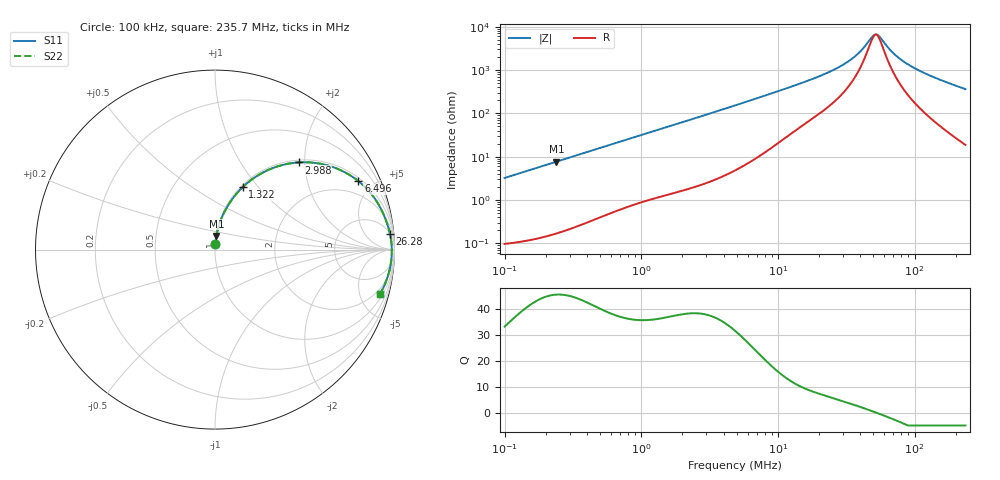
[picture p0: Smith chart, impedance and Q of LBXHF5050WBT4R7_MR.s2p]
! LBXHF5050WBT4R7_MR  S-PARAMETER MODEL  ( General Type )
! Model Generated by TAIYO YUDEN Corporation (http://www.ty-top.com)
! Version 1.0
! TAIYO YUDEN Control No. 210719NI43SB-FBB
! Copyright(c) 2021 TAIYO YUDEN CO.,LTD. All Rights Reserved.
! Product Description (link to TY-COMPAS)
! https://ds.yuden.co.jp/TYCOMPAS/or/detail?pn=LBXHF5050WBT4R7MMR&u=M
! Products Name : Inductors
! Characteristics :
!  Inductance : 4.7 uH , SRF(min) : 35 MHz , DC Resistance(max) : 0.0696 Ohm
!  Rated Current : Saturation :2100 mA , Temp Rise : 1500 mA
!  Case Size : 5.0 x 5.0 / 0.197 x 0.197 [mm/inch] , Thickness : 2.2 / 0.087 [mm/inch]
!  (Conditions: Temperature = 25 degC , DC Bias Current/Voltage = 0A / 0V)
! External Node Assignments :
!  1  o---GGG---o  2
! GND o---------o GND
! Frequency Range : 0.1MHz  -  235.669543MHz  [ 402 STEP ]
# MHz S RI R 50
! Freq[MHz].  S11 Real  S11 Imag  S21 Real  S21 Imag  S12 Real  S12 Imag  S22 Real  S22 Imag
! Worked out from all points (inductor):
!   401 points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, 100 kHz to 235.7 MHz, reference 50 ohm
!   read as one part in series: L = 5.14 uH near 104 kHz
!   highest Q = 45.6 at 239.5 kHz (marker M1), where L = 5.13 uH
!   self-resonance near 51.84 MHz
!   S11 on the Smith chart (normalised r, x): 100 kHz: 1.00, +0.06; 1.322 MHz: 1.02, +0.83; 2.988 MHz: 1.05, +1.87; 6.496 MHz: 1.16, +4.11; 26.28 MHz: 5, +21; 235.7 MHz: 1.38, -7.25
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0.1  0.00201 0.0322  0.998 -0.0322  0.998 -0.0322  0.00201 0.0322
0.239543  0.00758 0.0765  0.9924 -0.0765  0.9924 -0.0765  0.00758 0.0765
0.367165  0.0163 0.1157  0.9837 -0.1157  0.9837 -0.1157  0.0163 0.1157
0.767767  0.0617 0.2272  0.9383 -0.2272  0.9383 -0.2272  0.0617 0.2272
1.322181  0.154 0.3474  0.846 -0.3474  0.846 -0.3474  0.154 0.3474
1.348099  0.1588 0.352  0.8412 -0.352  0.8412 -0.352  0.1588 0.352
1.949423  0.2761 0.4341  0.7239 -0.4341  0.7239 -0.4341  0.2761 0.4341
2.988015  0.4662 0.4858  0.5338 -0.4858  0.5338 -0.4858  0.4662 0.4858
4.854581  0.6933 0.4456  0.3067 -0.4456  0.3067 -0.4456  0.6933 0.4456
6.495508  0.7993 0.3812  0.2007 -0.3812  0.2007 -0.3812  0.7993 0.3812
10.15127  0.9011 0.268  0.0989 -0.268  0.0989 -0.268  0.9011 0.268
17.8243  0.957 0.1507  0.043 -0.1507  0.043 -0.1507  0.957 0.1507
26.28014  0.9746 0.0893  0.0254 -0.0893  0.0254 -0.0893  0.9746 0.0893
31.91063  0.9797 0.0623  0.0203 -0.0623  0.0203 -0.0623  0.9797 0.0623
37.27189  0.9825 0.042  0.0175 -0.042  0.0175 -0.042  0.9825 0.042
50.84796  0.9851 0.00307  0.0149 -0.00307  0.0149 -0.00307  0.9851 0.00307
54.95365  0.9852 -0.00654  0.0148 0.00654  0.0148 0.00654  0.9852 -0.00654
65.44454  0.9847 -0.0284  0.0153 0.0284  0.0153 0.0284  0.9847 -0.0284
79.46593  0.9827 -0.0537  0.0173 0.0537  0.0173 0.0537  0.9827 -0.0537
104.2825  0.9771 -0.0924  0.0229 0.0924  0.0229 0.0924  0.9771 -0.0924
150.7981  0.9612 -0.1543  0.0388 0.1543  0.0388 0.1543  0.9612 -0.1543
235.6695  0.9185 -0.249  0.0815 0.249  0.0815 0.249  0.9185 -0.249
